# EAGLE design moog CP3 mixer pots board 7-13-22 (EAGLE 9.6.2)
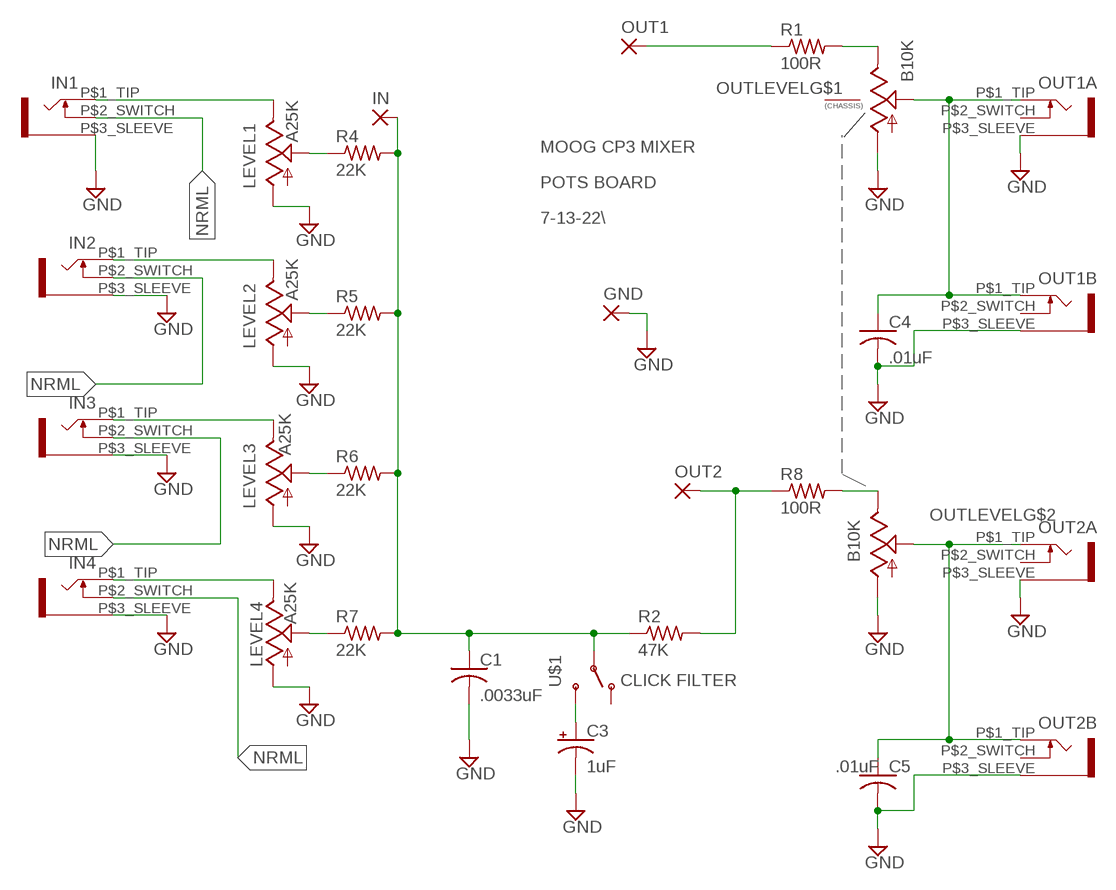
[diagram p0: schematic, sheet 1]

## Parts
C1  .0033uF  C-US025-030X050  [C025-030X050]
C3  1uF  CPOL-USE2,5-6E  [E2,5-6E]
C4  .01uF  C-US025-030X050  [C025-030X050]
C5  .01uF  C-US025-030X050  [C025-030X050]
GND  WIREPAD1,6/0,9  [1,6/0,9]
IN  WIREPAD1,6/0,9  [1,6/0,9]
IN1  WQP-PJ301M-12_JACK  [WQP-PJ301M-12_JACK]
IN2  WQP-PJ301M-12_JACK  [WQP-PJ301M-12_JACK]
IN3  WQP-PJ301M-12_JACK  [WQP-PJ301M-12_JACK]
IN4  WQP-PJ301M-12_JACK  [WQP-PJ301M-12_JACK]
LEVEL1  A25K  9MM_SNAP-IN_POT_  [9MM_SNAP-IN_POT]
LEVEL2  A25K  9MM_SNAP-IN_POT_  [9MM_SNAP-IN_POT]
LEVEL3  A25K  9MM_SNAP-IN_POT_  [9MM_SNAP-IN_POT]
LEVEL4  A25K  9MM_SNAP-IN_POT_  [9MM_SNAP-IN_POT]
OUT1  1,6/0,9  [1,6/0,9]
OUT1A  WQP-PJ301M-12_JACK  [WQP-PJ301M-12_JACK]
OUT1B  WQP-PJ301M-12_JACK  [WQP-PJ301M-12_JACK]
OUT2  1,6/0,9  [1,6/0,9]
OUT2A  WQP-PJ301M-12_JACK  [WQP-PJ301M-12_JACK]
OUT2B  WQP-PJ301M-12_JACK  [WQP-PJ301M-12_JACK]
OUTLEVEL  B10K  ALPHA-9MM-DUALPOT  [DUAL_9MM_SNAP-IN_POT]
R1  100R  R-US_0204/7  [0204/7]
R2  47K  R-US_0204/7  [0204/7]
R4  22K  R-US_0204/7  [0204/7]
R5  22K  R-US_0204/7  [0204/7]
R6  22K  R-US_0204/7  [0204/7]
R7  22K  R-US_0204/7  [0204/7]
R8  100R  R-US_0204/7  [0204/7]
U$1  CLICK FILTER  SUBMINI_SPDT  [SUBMINI_TOGGLE]

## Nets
GND: C1.2 C3.- C4.2 C5.2 GND.1(P) IN1.P$3_SLEEVE IN2.P$3_SLEEVE IN3.P$3_SLEEVE IN4.P$3_SLEEVE LEVEL1.1(A) LEVEL2.1(A) LEVEL3.1(A) LEVEL4.1(A) OUT1A.P$3_SLEEVE OUT1B.P$3_SLEEVE OUT2A.P$3_SLEEVE OUT2B.P$3_SLEEVE OUTLEVEL.1(A) OUTLEVEL.1B(A)
N$1: C1.1 IN.1(P) R2.1 R4.2 R5.2 R6.2 R7.2 U$1.COM(COMMON)
N$2: LEVEL1.2(S) R4.1
N$3: LEVEL2.2(S) R5.1
N$4: LEVEL3.2(S) R6.1
N$5: LEVEL4.2(S) R7.1
N$6: IN1.P$1_TIP LEVEL1.3(E)
N$7: IN2.P$1_TIP LEVEL2.3(E)
N$8: IN3.P$1_TIP LEVEL3.3(E)
N$9: IN4.P$1_TIP LEVEL4.3(E)
N$10: OUT1.1(P) R1.1
N$11: C3.+ U$1.3(S)
N$13: OUTLEVEL.3(E) R1.2
N$14: C4.1 OUT1A.P$1_TIP OUT1B.P$1_TIP OUTLEVEL.2(S)
N$15: OUT2.1(P) R2.2 R8.1
N$16: OUTLEVEL.3B(E) R8.2
N$17: C5.1 OUT2A.P$1_TIP OUT2B.P$1_TIP OUTLEVEL.2B(S)
NRML: IN1.P$2_SWITCH IN2.P$2_SWITCH IN3.P$2_SWITCH IN4.P$2_SWITCH
Unconnected: OUT1A.P$2_SWITCH OUT1B.P$2_SWITCH OUT2A.P$2_SWITCH OUT2B.P$2_SWITCH OUTLEVEL.CHASSIS1 OUTLEVEL.CHASSIS2 U$1.1(O)

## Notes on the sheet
- MOOG CP3 MIXER
- POTS BOARD
- 7-13-22\

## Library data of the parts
C1 C4 C5 = rcl:C-US: CAPACITOR, American symbol; SPICEPREFIX: C
C3 = adafruit:CPOL-US: POLARIZED CAPACITOR, American symbol
GND IN = wirepad:WIREPAD: Wire PAD connect wire on PCB
IN1-IN4 OUT1A OUT1B OUT2A OUT2B = MusicThingModular:WQP-PJ301M-12_JACK
LEVEL1-LEVEL4 = MusicThingModular:9MM_SNAP-IN_POT: 9mm vertical snap-in pot, Alpha / Panasonic style
OUT1 OUT2 = wirepad:1,6/0,9: THROUGH-HOLE PAD
OUTLEVEL = MusicThingModular:ALPHA-9MM-DUALPOT: 9mm vertical snap-in pot, Alpha / Panasonic style, with a connection to the metal chassis for grounding
R1 R2 R4-R8 = rcl:R-US_: RESISTOR, American symbol
U$1 = MusicThingModular-CL:SUBMINI_SPDT

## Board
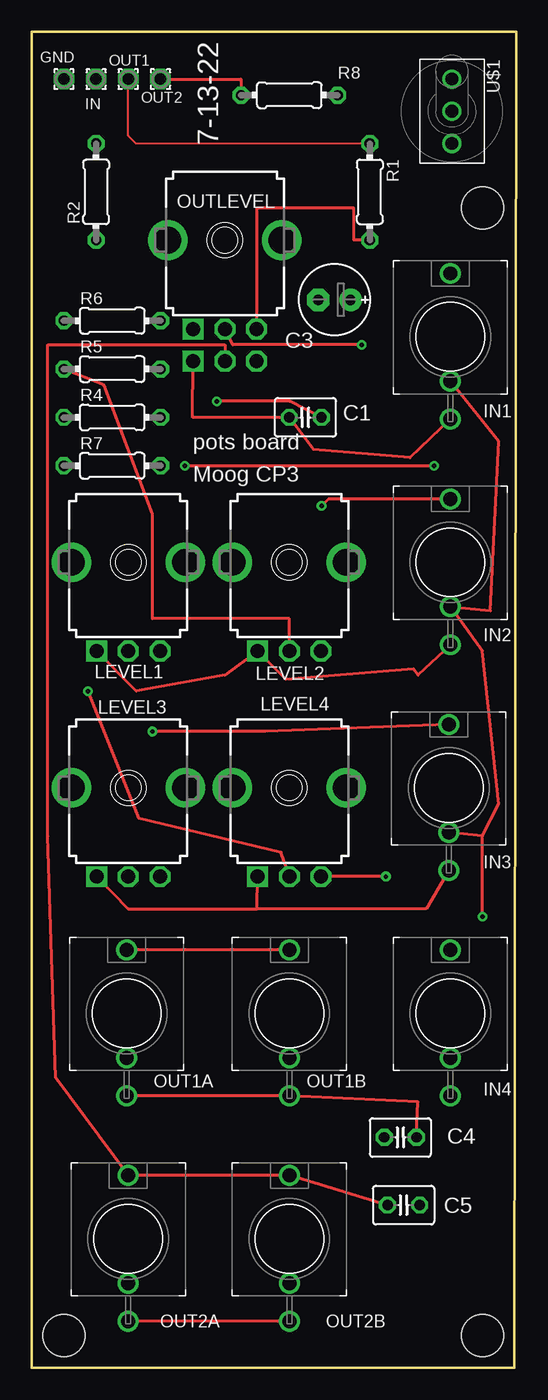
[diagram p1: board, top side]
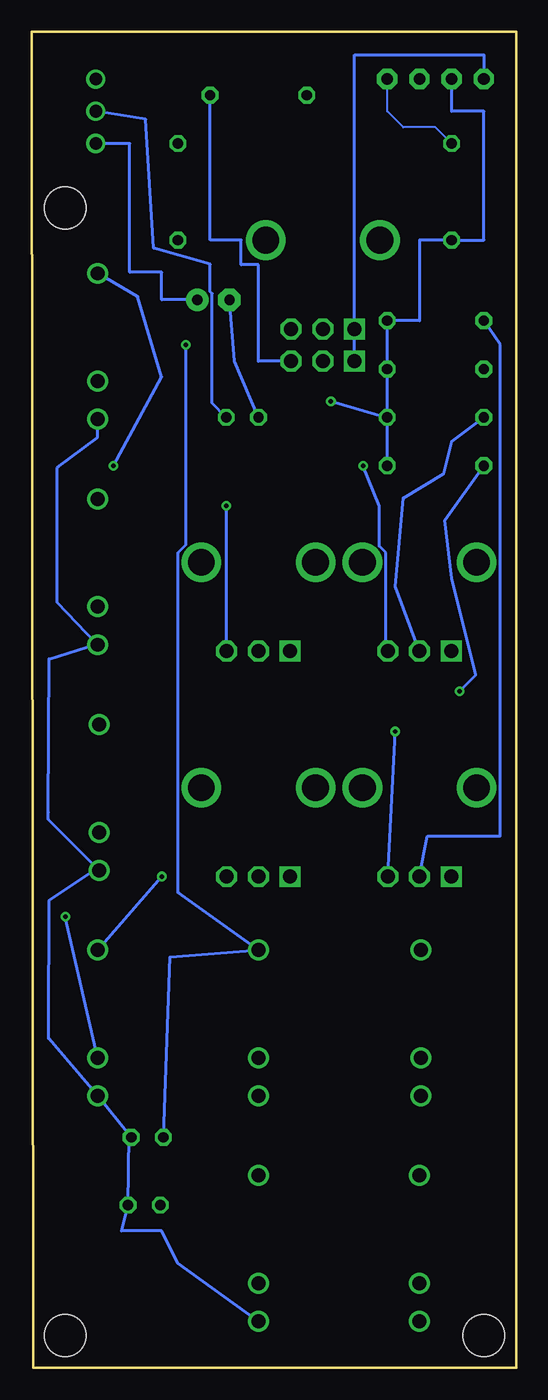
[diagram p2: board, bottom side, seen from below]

Size 38.21 x 105.33 mm. Coordinates in mm from the lower left corner, seen from the top.
Outline: 0,0 38.08,0 38.21,105.33 0,105.33 0,0
Copper layers (1*16): Top 0.035mm / dielectric 1.5mm / Bottom 0.035mm
Design rules "default": minimum track width 6mil, minimum drill 0.35mm, track to track 6mil, track to pad 6mil, pad to pad 6mil, via to via 6mil, smd to smd 6mil, copper to edge 40mil, drill to drill 6mil, minimum pad ring 10mil, minimum via ring 8mil, stop-mask expansion 4mil, vias tented up to drill 0mil, thermal gap 10mil
Holes 3.3 mm at 2.54,2.54 35.56,2.54 35.56,91.44

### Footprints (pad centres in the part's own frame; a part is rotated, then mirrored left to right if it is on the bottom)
C025-030X050 = drill 0.813 octagon: 1 -1.27,0; 2 1.27,0
E2,5-6E = drill 0.813 pad 1.778: + -1.27,0 | drill 0.813 pad 1.778 octagon: - 1.27,0
1,6/0,9 = drill 0.914 pad 1.6 octagon: 1 0,0
WQP-PJ301M-12_JACK = drill 1.1: P$1_TIP 0,5; P$2_SWITCH 0,-3.5; P$3_SLEEVE 0,-6.5
9MM_SNAP-IN_POT = drill 1.1 square: 1 -2.5,-7 | drill 1.1 octagon: 2 0,-7; 3 2.5,-7 | drill 2.1 pad 2.794: CHASSIS1 -4.5,0; CHASSIS2 4.5,0
DUAL_9MM_SNAP-IN_POT = drill 1.1 square: 1 -2.5,-7; 1B -2.5,-9.54 | drill 1.1 octagon: 2 0,-7; 2B 0,-9.54; 3 2.5,-7; 3B 2.5,-9.54 | drill 2.1 pad 2.54: CHASSIS1 -4.5,0; CHASSIS2 4.5,0
0204/7 = drill 0.813 octagon: 1 -3.81,0; 2 3.81,0
SUBMINI_TOGGLE = drill 1 pad 1.422: 1 -2.54,0; 3 2.54,0; COM 0,0

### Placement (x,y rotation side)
C1  21.59,74.93 180 top
C3  23.88,84.2 180 top
C4  29.08,18.16 0 top
C5  29.34,12.83 0 top
GND  2.54,101.6 0 top
IN  5.08,101.6 0 top
IN1  33.02,81.28 0 top
IN2  33.02,63.5 0 top
IN3  32.89,45.72 0 top
IN4  33.02,27.94 0 top
LEVEL1  7.62,63.5 0 top
LEVEL2  20.32,63.5 0 top
LEVEL3  7.62,45.72 0 top
LEVEL4  20.32,45.72 0 top
OUT1  7.62,101.6 0 top
OUT1A  7.49,27.94 0 top
OUT1B  20.32,27.94 0 top
OUT2  10.16,101.6 0 top
OUT2A  7.62,10.16 0 top
OUT2B  20.32,10.16 0 top
OUTLEVEL  15.24,88.9 0 top
R1  26.67,92.71 270 top
R2  5.08,92.71 90 top
R4  6.35,74.93 0 top
R5  6.35,78.74 0 top
R6  6.35,82.55 0 top
R7  6.35,71.12 0 top
R8  20.32,100.33 0 top
U$1  33.15,99.06 270 top

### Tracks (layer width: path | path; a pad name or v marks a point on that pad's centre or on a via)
GND
  Top 0.254: IN3.P$3_SLEEVE 31.11,36.2 17.78,36.2 | 17.78,36.2 LEVEL4.1 | LEVEL3.1 7.62,36.2 17.78,36.2 | IN2.P$3_SLEEVE 30.48,54.61 30.12,55.11 20.05,54.27 LEVEL2.1 15.24,54.61 8.26,53.34 LEVEL1.1 | IN1.P$3_SLEEVE 29.84,71.75 22.23,72.39 C1.2 12.7,74.93 OUTLEVEL.1B | OUT1A.P$3_SLEEVE OUT1B.P$3_SLEEVE 30.48,20.95 C4.2 | OUT2B.P$3_SLEEVE OUT2A.P$3_SLEEVE
  Bottom 0.254: GND.1 2.54,103.5 12.74,103.5 OUTLEVEL.1 OUTLEVEL.1B | C1.2 22.23,79.38 C3.- | IN2.P$3_SLEEVE 33.09,57.08 | 33.09,57.08 36.2,60.33 36.2,70.96 33.02,73.35 IN1.P$3_SLEEVE | IN3.P$3_SLEEVE 33.03,39.36 | 33.03,39.36 36.89,43.23 36.89,43.82 36.83,55.88 33.09,57.08 | C4.2 30.53,18.38 | 30.53,18.38 IN4.P$3_SLEEVE 36.87,25.97 36.87,26.67 36.83,36.83 33.03,39.36 | 30.53,18.38 C5.2 31.11,10.79 27.94,10.79 26.67,8.26 OUT2B.P$3_SLEEVE
N$1  (via drill 0.35)
  Top 0.254: C1.1 20.32,76.2 v14.61,76.2
  Bottom 0.254: IN.1 5.08,99.06 2.54,99.06 2.54,88.9 R2.1 7.62,88.9 7.62,82.55 R6.2 R5.2 R4.2 | R7.2 R4.2 | C1.1 23.98,76.05 23.98,84.69 24.13,84.84 24.13,87 28.57,88.27 29.21,98.42 U$1.COM | v14.61,76.2 R4.2
N$2
  Bottom 0.254: R4.1 5.08,73.03 5.71,70.48 8.89,68.58 9.53,61.59 LEVEL1.2
N$3
  Top 0.254: LEVEL2.2 20.32,59.05 9.53,59.05 9.53,67.31 5.71,77.47 R5.1
N$4
  Bottom 0.254: LEVEL3.2 6.99,41.91 1.25,41.91 1.25,80.64 R6.1
N$5  (via drill 0.35)
  Top 0.254: LEVEL4.2 19.68,40.64 8.46,43.31 v4.45,53.34
  Bottom 0.254: v4.45,53.34 3.17,54.61 5.08,62.23 5.62,66.81 R7.1
N$6  (via drill 0.35)
  Top 0.254: v12.06,71.12 v31.75,71.12
  Bottom 0.254: LEVEL1.3 10.28,56.66 10.28,64.26 10.79,64.77 10.79,67.94 v12.06,71.12 | v31.75,71.12 27.94,78.11 29.84,84.45 IN1.P$1_TIP
N$7  (via drill 0.35)
  Top 0.254: IN2.P$1_TIP 23.41,68.5 v22.86,67.94
  Bottom 0.254: LEVEL2.3 22.86,56.5 v22.86,67.94
N$8  (via drill 0.35)
  Top 0.254: IN3.P$1_TIP 18.41,50.16 v9.53,50.16
  Bottom 0.254: LEVEL3.3 v9.53,50.16
N$9  (via drill 0.35)
  Top 0.254: v27.94,38.73 LEVEL4.3
  Bottom 0.254: IN4.P$1_TIP v27.94,38.73
N$10
  Top 0.152: R1.1 8.26,96.52 7.62,97.16 OUT1.1
N$11
  Bottom 0.254: C3.+ 27.94,84.2 27.94,86.36 30.48,86.36 30.48,96.52 U$1.3
N$13
  Top 0.254: R1.2 25.4,88.9 25.4,91.44 17.74,91.44 OUTLEVEL.3
N$14  (via drill 0.35)
  Top 0.254: OUT1B.P$1_TIP OUT1A.P$1_TIP | OUTLEVEL.2 15.88,80.64 v26.04,80.64
  Bottom 0.254: C4.1 27.3,32.38 OUT1B.P$1_TIP 26.67,37.47 26.66,37.48 26.66,64.26 26.04,64.88 v26.04,80.64
N$15
  Top 0.254: OUT2.1 16.51,101.6 R8.1
  Bottom 0.152: R2.2 6.35,97.79 8.89,97.79 10.16,99.06 OUT2.1
N$16
  Bottom 0.254: OUTLEVEL.3B 20.32,79.36 20.32,86.96 21.68,86.96 21.68,88.9 24.13,88.9 R8.2
N$17
  Top 0.254: C5.1 OUT2B.P$1_TIP OUT2A.P$1_TIP 1.91,22.86 1.27,41.91 1.27,80.64 15.24,80.64 OUTLEVEL.2B
NRML  (via drill 0.35)
  Top 0.254: v35.56,35.56 35.56,41.91 | 35.56,41.91 IN3.P$2_SWITCH | 35.56,41.91 36.83,44.45 35.56,56.52 IN2.P$2_SWITCH 36.2,59.69 36.83,73.03 IN1.P$2_SWITCH
  Bottom 0.254: IN4.P$2_SWITCH v35.56,35.56

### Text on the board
tNames: 7-13-22 | pots board | Moog CP3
